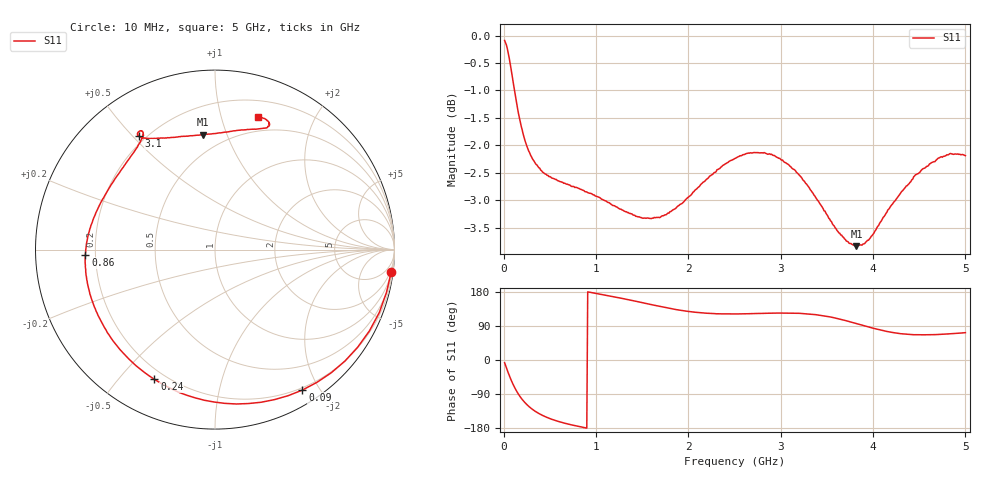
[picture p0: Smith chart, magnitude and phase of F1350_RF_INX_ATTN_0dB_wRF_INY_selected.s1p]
! S-parameters for RF_INX input IDT F1350 DPD Demodulator
! Date Measured:  2015-11-25  RGG
!  Port 1 = Pin 35 = RF_INX
! STATE: RF_INY selected, 0 dB attenuation (Gain = Gmax - 0 dB)
! RF Frequency:  10 MHz to 5000 MHz
! RF_INY, IF_I+, IF_I-, IF_Q+, and IF_Q- terminated
! 2300 MHz, 0 dBm signal applied to LO_IN
! Vcc = +5.00 Volts  Icc = approx 275 mA.
! NOTES:  The device was measured on a custom printed circuit evaluation board with individual 50 ohm
!  microstrip lines to the RF and LO pins. The 50 ohm microstrip lines were de-embedded using reference
!  plane extensions
! Instrument Manufacturer:  Agilent Technologies
! Instrument Model:  E5071C
! Instrument Serial Number:  MY46419053
! Instrument Firmware Rev:  A.11.31
! Frequency Re{S11} Im{S11}
# HZ  S  RI R 50.00
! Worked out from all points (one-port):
!   500 points, 10 MHz to 5 GHz, reference 50 ohm
!   lowest |S11| = -3.8 dB at 3.82 GHz (marker M1), VSWR 4.60, Z = 19 + j41.3 ohm
!   |S11| at or under -10 dB: nowhere
!   S11 on the Smith chart (normalised r, x): 10 MHz: 1, -16; 90 MHz: 0.17, -1.79; 240 MHz: 0.16, -0.63; 860 MHz: 0.16, -0.02; 3.1 GHz: 0.17, +0.52; 5 GHz: 0.35, +1.31
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1e7  0.9821 -0.1234
2e7  0.9551 -0.2401
4e7  0.8604 -0.453
6e7  0.7244 -0.6208
9e7  0.4873 -0.7822
1.2e8  0.2564 -0.8506
1.6e8  -0.00398 -0.8494
2e8  -0.1976 -0.7968
2.4e8  -0.3374 -0.723
3.1e8  -0.4965 -0.5922
3.9e8  -0.6 -0.4621
5e8  -0.672 -0.3194
6.4e8  -0.7114 -0.1848
8.6e8  -0.7224 -0.0287
1.26e9  -0.6665 0.1965
1.89e9  -0.4701 0.5183
2.19e9  -0.4088 0.6155
2.51e9  -0.4044 0.6589
3.1e9  -0.4242 0.6311
3.13e9  -0.4194 0.6293
3.43e9  -0.3297 0.6195
3.76e9  -0.1137 0.6365
3.82e9  -0.0671 0.6395
4.17e9  0.1873 0.6691
4.38e9  0.2776 0.677
4.52e9  0.3027 0.6901
4.69e9  0.2992 0.7106
5e9  0.2387 0.7399
